(* Logix 5000 AddOnInstructionDefinition export AMCI_NXFE2_Run_Blend_Move; software revision 20.03 *)

ADD_ON_INSTRUCTION AMCI_NXFE2_Run_Blend_Move   (* revision 1.0, vendor AMCI, ExecuteEnableInFalse *)
VAR_INPUT
   Axis_Status_bits : INT; {required}
   Direction_0_for_CW_1_for_CCW : BOOL; {required}
END_VAR
VAR_IN_OUT
   NXFE2_output_data : _000A:NXFE2_0986AEB4:O:0; {required}
END_VAR
VAR_OUTPUT
   EN : BOOL; {access Read Only, visible}
   ER : BOOL; {access Read Only, visible}
END_VAR
VAR
   command_data_block : INT[10];
        [0]   // Command Bits MSW
        [1]   // Command Bits LSW
        [2]   // Upper Target Position
        [3]   // Lower Target Position
        [4]   // Upper Programmed Speed
        [5]   // Lower Programmed Speed
END_VAR

ROUTINE EnableInFalse   (* ladder *)
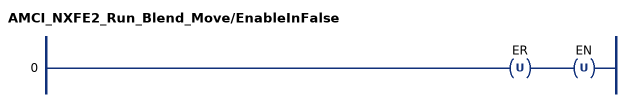
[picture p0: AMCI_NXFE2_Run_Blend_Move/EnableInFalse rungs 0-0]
   0: OTU(ER)OTU(EN);
END_ROUTINE

ROUTINE Logic   (* ladder *)
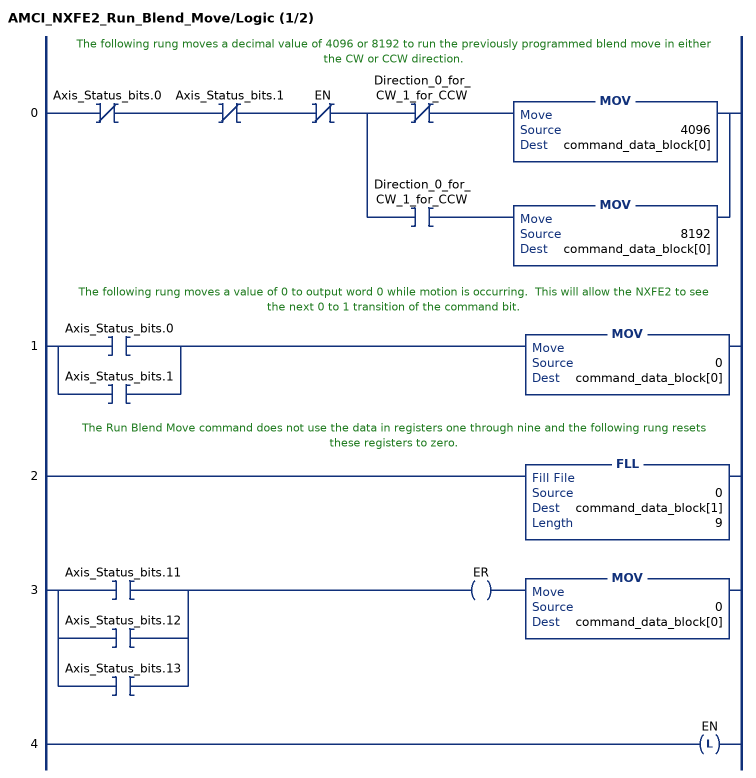
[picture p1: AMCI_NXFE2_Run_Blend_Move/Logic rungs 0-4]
   // The following rung moves a decimal value of 4096 or 8192 to run the previously programmed blend move in either the CW or CCW direction.
   0: XIO(Axis_Status_bits.0)XIO(Axis_Status_bits.1)XIO(EN)[XIO(Direction_0_for_CW_1_for_CCW) MOV(4096,command_data_block[0]) ,XIC(Direction_0_for_CW_1_for_CCW) MOV(8192,command_data_block[0]) ];
   // The following rung moves a value of 0 to output word 0 while motion is occurring.  This will allow the NXFE2 to see the next 0 to 1 transition of the command bit.
   1: [XIC(Axis_Status_bits.0) ,XIC(Axis_Status_bits.1) ]MOV(0,command_data_block[0]);
   // The Run Blend Move command does not use the data in registers one through nine and the following rung resets these registers to zero.
   2: FLL(0,command_data_block[1],9);
   3: [XIC(Axis_Status_bits.11) ,XIC(Axis_Status_bits.12) ,XIC(Axis_Status_bits.13) ]OTE(ER)MOV(0,command_data_block[0]);
   4: OTL(EN);
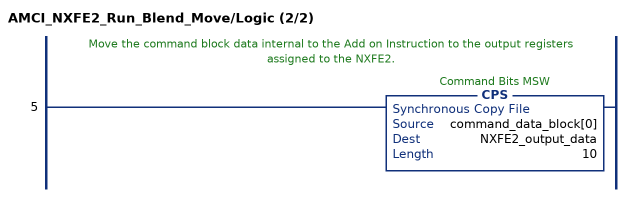
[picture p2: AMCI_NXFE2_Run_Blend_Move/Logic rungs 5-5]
   // Move the command block data internal to the Add on Instruction to the output registers assigned to the NXFE2.
   5: CPS(command_data_block[0],NXFE2_output_data,10);
END_ROUTINE
END_ADD_ON_INSTRUCTION
